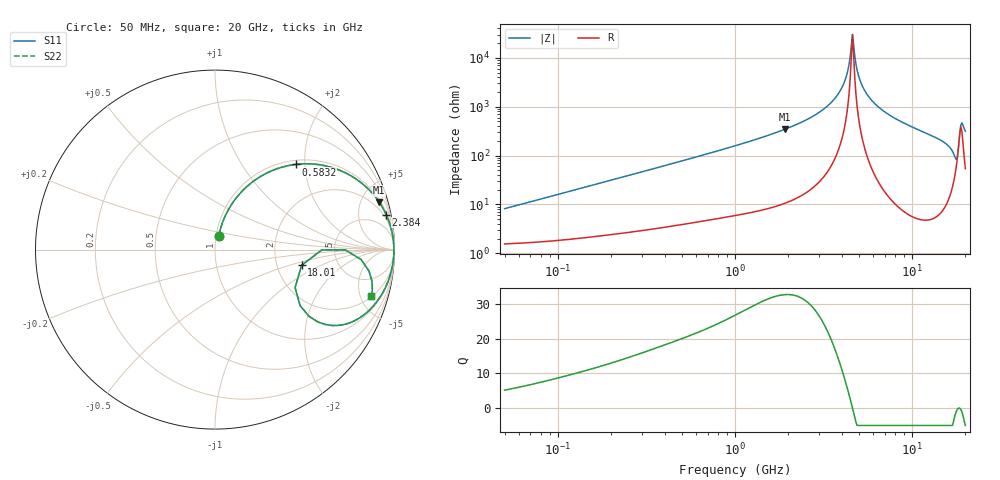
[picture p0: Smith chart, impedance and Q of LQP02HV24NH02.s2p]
!Murata Part Number: LQP02HV24NH02
!These Parameters are Measured in Series Mode Connection
!  o--[Z]--o
!Port1  Port2
!  o-------o
!Freq. Start=50[MHz] Stop=20[GHz], 401[Steps]
# Hz S RI R 50
!Freq.(Hz) S11(Real) S11(Imag) S21(Real) S21(Imag) S12(Real) S12(Imag) S22(Real) S22(Imag)
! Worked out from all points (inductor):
!   401 points, 50 MHz to 20 GHz, reference 50 ohm
!   read as one part in series: L = 25.5 nH near 51.52 MHz
!   highest Q = 32.7 at 1.904 GHz (marker M1), where L = 28.6 nH
!   self-resonance near 4.608 GHz
!   S11 on the Smith chart (normalised r, x): 50 MHz: 1.03, +0.16; 583.2 MHz: 1.08, +1.80; 2.384 GHz: 1.31, +9.68; 18.01 GHz: 2.75, -0.64; 20 GHz: 2.08, -6.20
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5e7  0.0214 0.0774  0.9786 -0.0774  0.9786 -0.0774  0.0214 0.0774
1.364002e8  0.0617 0.1978  0.9383 -0.1978  0.9383 -0.1978  0.0617 0.1978
3.721004e8  0.2612 0.4118  0.7388 -0.4118  0.7388 -0.4118  0.2612 0.4118
5.831961e8  0.4511 0.4747  0.5489 -0.4747  0.5489 -0.4747  0.4511 0.4747
1e9  0.7069 0.4369  0.2931 -0.4369  0.2931 -0.4369  0.7069 0.4369
1.904239e9  0.9146 0.2646  0.0854 -0.2646  0.0854 -0.2646  0.9146 0.2646
2.383959e9  0.9534 0.1955  0.0466 -0.1955  0.0466 -0.1955  0.9534 0.1955
2.728004e9  0.9699 0.1545  0.0301 -0.1545  0.0301 -0.1545  0.9699 0.1545
3.908127e9  0.9939 0.0481  0.00607 -0.0481  0.00607 -0.0481  0.9939 0.0481
4.212059e9  0.9958 0.0263  0.00422 -0.0263  0.00422 -0.0263  0.9958 0.0263
4.608136e9  0.9967 0.000122  0.00331 -0.000122  0.00331 -0.000122  0.9967 0.000122
4.748272e9  0.9967 -0.00862  0.00333 0.00862  0.00333 0.00862  0.9967 -0.00862
4.966507e9  0.9964 -0.0218  0.00365 0.0218  0.00365 0.0218  0.9964 -0.0218
5.352748e9  0.995 -0.0438  0.00499 0.0438  0.00499 0.0438  0.995 -0.0438
6.125241e9  0.9899 -0.0839  0.0101 0.0839  0.0101 0.0839  0.9899 -0.0839
7.442007e9  0.9758 -0.1439  0.0242 0.1439  0.0242 0.1439  0.9758 -0.1439
1.276073e10  0.8661 -0.3312  0.1339 0.3312  0.1339 0.3312  0.8661 -0.3312
1.621653e10  0.6807 -0.4228  0.3193 0.4228  0.3193 0.4228  0.6807 -0.4228
1.721783e10  0.5237 -0.3718  0.4763 0.3718  0.4763 0.3718  0.5237 -0.3718
1.800918e10  0.4822 -0.0876  0.5178 0.0876  0.5178 0.0876  0.4822 -0.0876
1.912117e10  0.8583 -0.1201  0.1417 0.1201  0.1417 0.1201  0.8583 -0.1201
2e10  0.8716 -0.2587  0.1284 0.2587  0.1284 0.2587  0.8716 -0.2587
